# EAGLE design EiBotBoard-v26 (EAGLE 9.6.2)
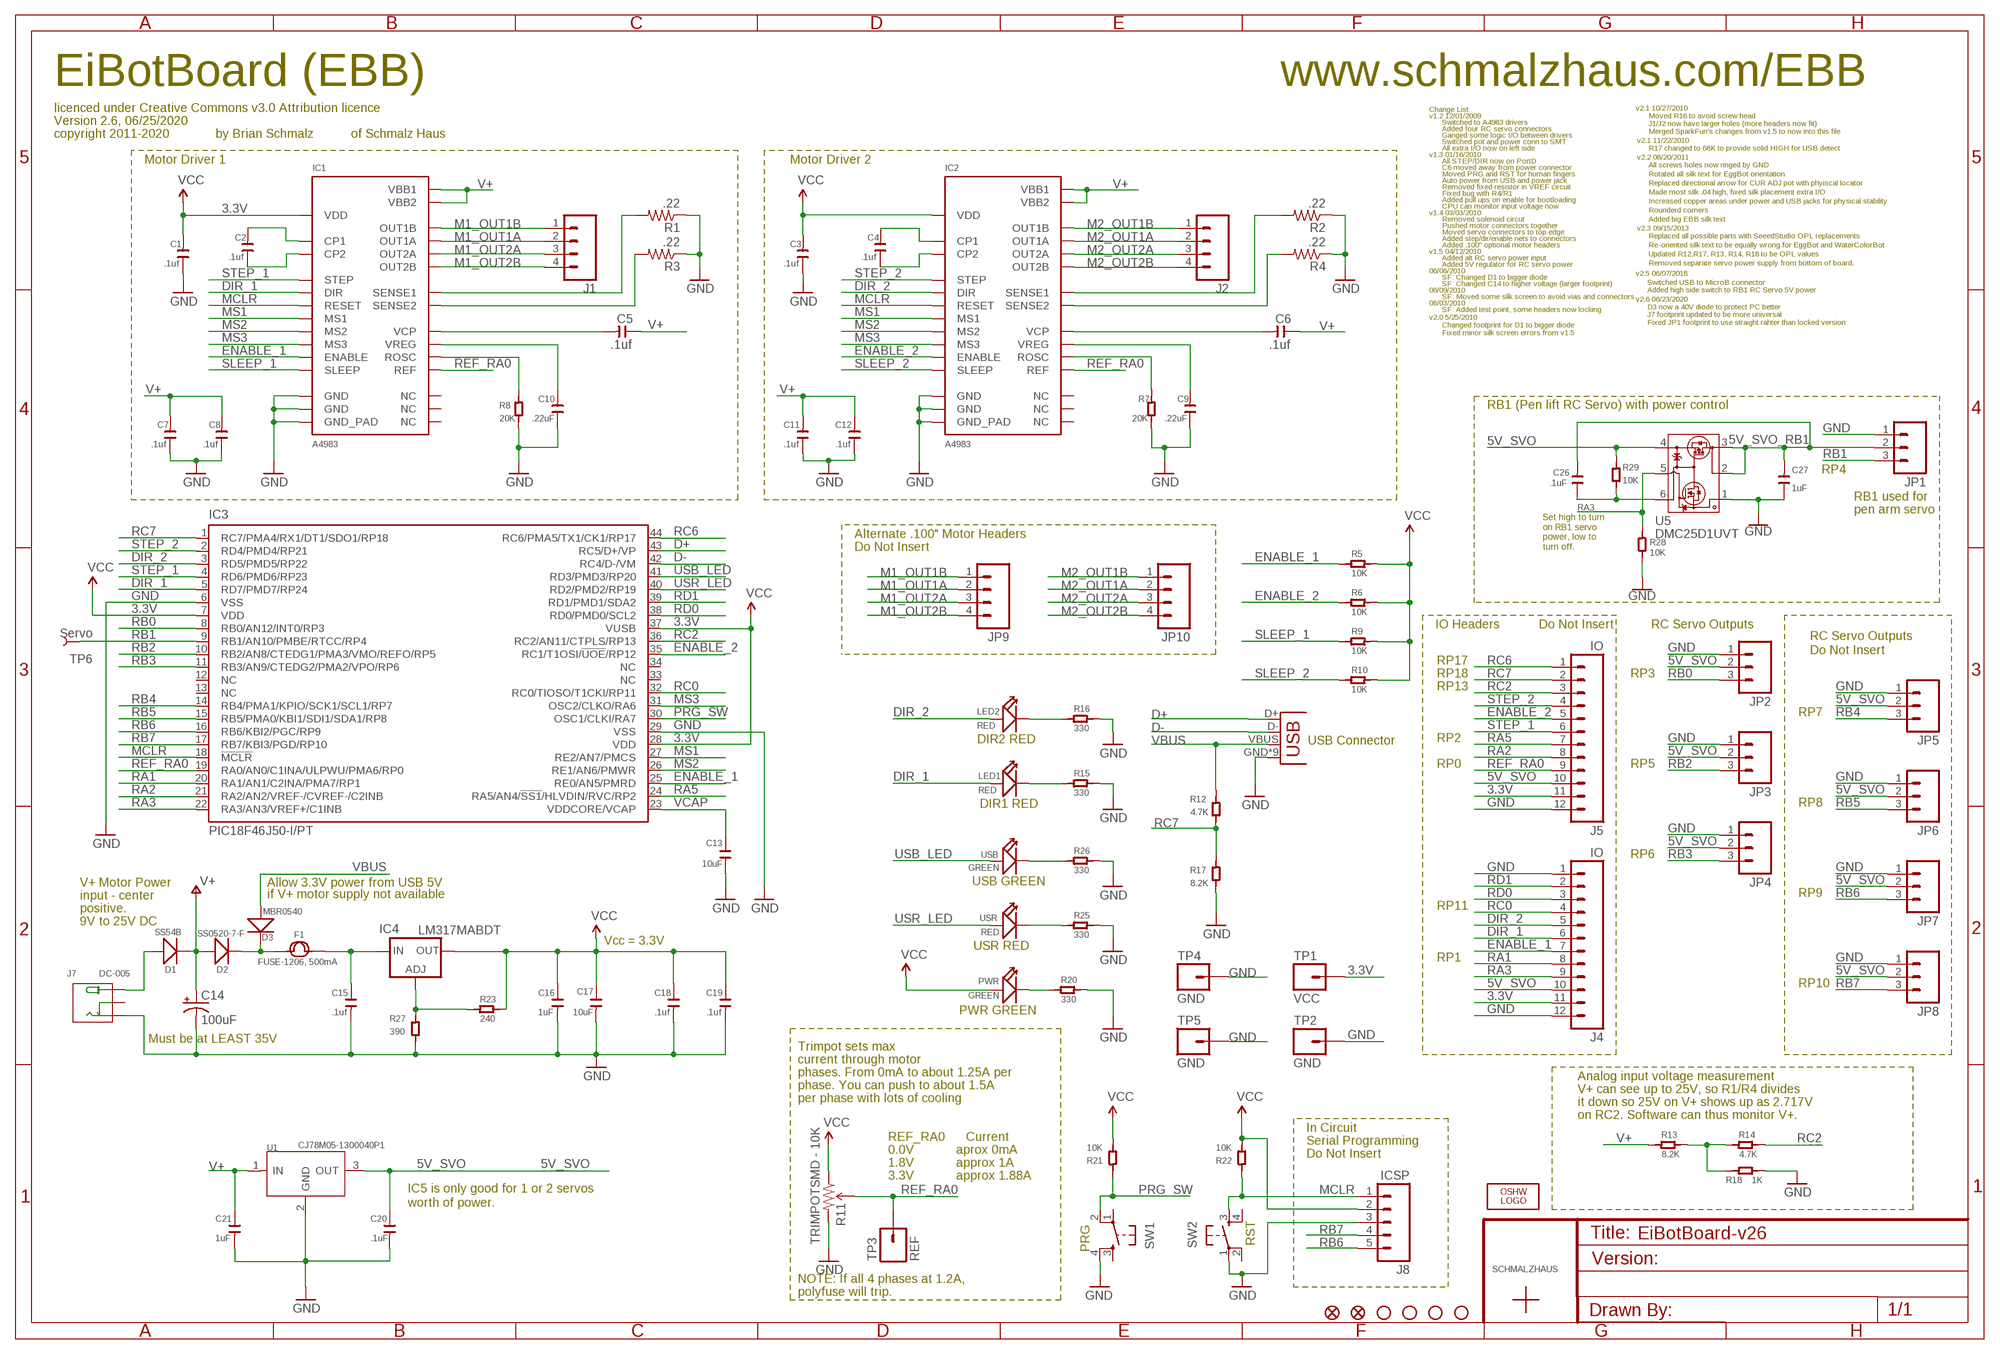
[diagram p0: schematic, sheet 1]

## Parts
C1  .1uf  C-0603  [C0603]
C2  .1uf  C-0603  [C0603]
C3  .1uf  C-0603  [C0603]
C4  .1uf  C-0603  [C0603]
C5  .1uf  C-0603  [C0603]
C6  .1uf  C-0603  [C0603]
C7  .1uf  C-0603  [C0603]
C8  .1uf  C-0603  [C0603]
C9  .22uF  C-0603  [C0603]
C10  .22uF  C-0603  [C0603]
C11  .1uf  C-0603  [C0603]
C12  .1uf  C-0603  [C0603]
C13  10uF  C-0805  [C0805]
C14  100uF  CAP_POLD  [PANASONIC_D]
C15  .1uf  C-0603  [C0603]
C16  1uF  C-0603  [C0603]
C17  10uF  C-0805  [C0805]
C18  .1uf  C-0603  [C0603]
C19  .1uf  C-0603  [C0603]
C20  .1uF  C-0603  [C0603]
C21  1uF  C-0603  [C0603]
C26  .1uF  C-0603  [C0603]
C27  1uF  C-0603  [C0603]
D1  SS54B  D-SMB  [SMB]
D2  SS0520-7-F  D-SOD-123  [SOD123]
D3  MBR0540  D-SOD-123  [SOD123]
F1  FUSE-1206, 500mA  FUSE-1206  [F1206]
IC1  A4983  [QFN28]
IC2  A4983  [QFN28]
IC3  PIC18F46J50-I/PT  PIC18F4J50  [TQFP44]
IC4  LM317MABDT  [DPACK]
J1  SCHMALZHAUS_M04  [SCHMALZHAUS_SCREWTERMINAL-3.5MM-4_LOCK]
J2  SCHMALZHAUS_M04  [SCHMALZHAUS_SCREWTERMINAL-3.5MM-4_LOCK]
J3  USBMICROB  [USB-MICROB_FCI_PINS]
J4  IO  M12PTH  [1X12]
J5  IO  M12PTH  [1X12]
J7  DC-005  CONN-POWER-JACK-2.1MM(DC-005)  [DCJ3P-14.2X11.0X9.0MM]
J8  ICSP  M05_WIDENOSILK  [1X05_NOSILK]
JP1  M031X03_NO_SILK  [1X03_NO_SILK]
JP2  M031X03_NO_SILK  [1X03_NO_SILK]
JP3  M031X03_NO_SILK  [1X03_NO_SILK]
JP4  M031X03_NO_SILK  [1X03_NO_SILK]
JP5  M031X03_NO_SILK  [1X03_NO_SILK]
JP6  M031X03_NO_SILK  [1X03_NO_SILK]
JP7  M031X03_NO_SILK  [1X03_NO_SILK]
JP8  M031X03_NO_SILK  [1X03_NO_SILK]
JP9  M04POLAR  [MOLEX-1X4]
JP10  M04POLAR  [MOLEX-1X4]
JP14  FIDUCIAL1X2  [FIDUCIAL-1X2]
JP15  FIDUCIAL1X2  [FIDUCIAL-1X2]
LED1  RED  LED  [LED0603]
LED2  RED  LED  [LED0603]
LOGO1  OSHW_LOGO_8MILX0100-NT  [OSHW_8X100_NOTEXT]
PWR  GREEN  LED  [LED0603]
R1  .22  R-US_R0805  [R0805]
R2  .22  R-US_R0805  [R0805]
R3  .22  R-US_R0805  [R0805]
R4  .22  R-US_R0805  [R0805]
R5  10K  R-0603  [R0603]
R6  10K  R-0603  [R0603]
R7  20K  R-0603  [R0603]
R8  20K  R-0603  [R0603]
R9  10K  R-0603  [R0603]
R10  10K  R-0603  [R0603]
R11  TRIMPOTSMD - 10K  TRIMPOTSMD  [TRIMPOT-3MM]
R12  4.7K  R-0603  [R0603]
R13  8.2K  R-0603  [R0603]
R14  4.7K  R-0603  [R0603]
R15  330  R-0603  [R0603]
R16  330  R-0603  [R0603]
R17  8.2K  R-0603  [R0603]
R18  1K  R-0603  [R0603]
R20  330  R-0603  [R0603]
R21  10K  R-0603  [R0603]
R22  10K  R-0603  [R0603]
R23  240  R-0603  [R0603]
R25  330  R-0603  [R0603]
R26  330  R-0603  [R0603]
R27  390  R-0603  [R0603]
R28  10K  R-0603  [R0603]
R29  10K  R-0603  [R0603]
SW1  PRG  TAC_SWITCHSND  [TACTILE_SWITCH_SMD]
SW2  RST  TAC_SWITCHSND  [TACTILE_SWITCH_SMD]
TP1  VCC  M01_WIDENOSLIK  [1X01_NOSILK]
TP2  GND  M01_WIDENOSLIK  [1X01_NOSILK]
TP3  REF  M01PTH  [1X01]
TP4  GND  M01_WIDENOSLIK  [1X01_NOSILK]
TP5  GND  M01_WIDENOSLIK  [1X01_NOSILK]
TP6  Servo  TEST-POINT3X5  [PAD.03X.05]
U1  CJ78M05-1300040P1  [TO252]
U5  DMC25D1UVT  [TSOT26]
U$1  SCHMALZHAUSSCHMALZHAUS_SMALL  [SCHMALZHAUS_SMALL]
U$2  STAND-OFF  [STAND-OFF]
U$3  STAND-OFF  [STAND-OFF]
U$4  STAND-OFF  [STAND-OFF]
U$5  STAND-OFF  [STAND-OFF]
USB  GREEN  LED  [LED0603]
USR  RED  LED  [LED0603]

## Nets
3.3V: C1.1 C3.1 C16.2 C17.2 C18.2 C19.2 IC1.P$15(VDD) IC2.P$15(VDD) IC3.7(VDD) IC3.28(VDD) IC3.37(VUSB) IC4.4(OUT) J4.11 J5.11 J8.2 PWR.+ R5.1 R6.1 R9.1 R10.1 R11.1(CCW) R21.2 R22.2 R23.2 TP1.1 ; supply symbol labelled VCC
5V_SVO: C20.2 J4.10 J5.10 JP2.2 JP3.2 JP4.2 JP5.2 JP6.2 JP7.2 JP8.2 R29.1 U1.3(OUT) U5.4(VIN_R1)
5V_SVO_RB1: C26.1 C27.1 JP1.2 U5.2(VOUT_C1$2) U5.3(VOUT_C1$1)
D+: IC3.43(RC5/D+/VP) J3.D+
D-: IC3.42(RC4/D-/VM) J3.D-
DIR_1: IC1.P$19(DIR) IC3.5(RD7/PMD7/RP24) J4.6 LED1.+
DIR_2: IC2.P$19(DIR) IC3.3(RD5/PMD5/RP22) J4.5 LED2.+
ENABLE_1: IC1.P$2(ENABLE) IC3.25(RE0/AN5/PMRD) J4.7 R5.2
ENABLE_2: IC2.P$2(ENABLE) IC3.35(RC1/T1OSI/!UOE!/RP12) J5.5 R6.2
GND: C1.2 C3.2 C7.2 C8.2 C9.2 C10.2 C11.2 C12.2 C13.1 C14.- C15.1 C16.1 C17.1 C18.1 C19.1 C20.1 C21.1 C27.2 IC1.P$3(GND) IC1.P$18(GND) IC1.P$29(GND_PAD) IC2.P$3(GND) IC2.P$18(GND) IC2.P$29(GND_PAD) IC3.6(VSS) IC3.29(VSS) J3.GND J3.GND@1(GND) J3.GND@2(GND) J3.GND@3(GND) J3.GND@4(GND) J3.GND@5(GND) J3.GND@6(GND) J3.GND@7(GND) J3.GND@8(GND) J4.1 J4.12 J5.12 J7.P$2(-) J8.3 JP1.1 JP2.1 JP3.1 JP4.1 JP5.1 JP6.1 JP7.1 JP8.1 R1.1 R2.1 R3.1 R4.1 R7.2 R8.2 R11.3(CW) R15.1 R16.1 R17.2 R18.2 R20.1 R25.1 R26.1 R27.2 R28.2 SW1.4 SW2.1 TP2.1 TP4.1 TP5.1 U1.2(GND) U5.1(R2)
M1_OUT1A: IC1.P$24(OUT1A) J1.2 JP9.2
M1_OUT1B: IC1.P$21(OUT1B) J1.1 JP9.1
M1_OUT2A: IC1.P$26(OUT2A) J1.3 JP9.3
M1_OUT2B: IC1.P$1(OUT2B) J1.4 JP9.4
M2_OUT1A: IC2.P$24(OUT1A) J2.2 JP10.2
M2_OUT1B: IC2.P$21(OUT1B) J2.1 JP10.1
M2_OUT2A: IC2.P$26(OUT2A) J2.3 JP10.3
M2_OUT2B: IC2.P$1(OUT2B) J2.4 JP10.4
MCLR: IC1.P$12(RESET) IC2.P$12(RESET) IC3.18(!MCLR!) J8.1 R22.1 SW2.3
MS1: IC1.P$9(MS1) IC2.P$9(MS1) IC3.27(RE2/AN7/PMCS)
MS2: IC1.P$10(MS2) IC2.P$10(MS2) IC3.26(RE1/AN6/PMWR)
MS3: IC1.P$11(MS3) IC2.P$11(MS3) IC3.31(OSC2/CLKO/RA6)
N$1: LED2.- R16.2
N$2: D2.- D3.- F1.1
N$3: C2.1 IC1.P$4(CP1)
N$4: R13.2 R14.1 R18.1
N$5: C2.2 IC1.P$5(CP2)
N$6: D1.+ J7.P$1(+)
N$7: LED1.- R15.2
N$8: R26.2 USB.-
N$9: IC4.1(ADJ) R23.1 R27.1
N$10: R25.2 USR.-
N$11: PWR.- R20.2
N$16: C4.1 IC2.P$4(CP1)
N$17: C4.2 IC2.P$5(CP2)
N$19: IC1.P$13(ROSC) R8.1
N$20: C10.1 IC1.P$8(VREG)
N$21: C5.1 IC1.P$6(VCP)
N$31: IC1.P$27(SENSE2) R3.2
N$32: IC1.P$23(SENSE1) R1.2
N$36: C15.2 F1.2 IC4.3(IN)
N$41: C6.1 IC2.P$6(VCP)
N$43: IC2.P$23(SENSE1) R2.2
N$44: IC2.P$27(SENSE2) R4.2
N$45: C9.1 IC2.P$8(VREG)
N$48: IC2.P$13(ROSC) R7.1
N$1234: C26.2 R29.2 U5.6(R1_C1)
PRG_SW: IC3.30(OSC1/CLKI/RA7) R21.1 SW1.2
RA1: IC3.20(RA1/AN1/C2INA/PMA7/RP1) J4.8
RA2: IC3.21(RA2/AN2/VREF-/CVREF-/C2INB) J5.8
RA3: IC3.22(RA3/AN3/VREF+/C1INB) J4.9 R28.1 U5.5(ON/OFF)
RA5: IC3.24(RA5/AN4/!SS1!/HLVDIN/RVC/RP2) J5.7
RB0: IC3.8(RB0/AN12/INT0/RP3) JP2.3
RB1: IC3.9(RB1/AN10/PMBE/RTCC/RP4) JP1.3 TP6.P$1
RB2: IC3.10(RB2/AN8/CTEDG1/PMA3/VMO/REFO/RP5) JP3.3
RB3: IC3.11(RB3/AN9/CTEDG2/PMA2/VPO/RP6) JP4.3
RB4: IC3.14(RB4/PMA1/KPIO/SCK1/SCL1/RP7) JP5.3
RB5: IC3.15(RB5/PMA0/KBI1/SDI1/SDA1/RP8) JP6.3
RB6: IC3.16(RB6/KBI2/PGC/RP9) J8.5 JP7.3
RB7: IC3.17(RB7/KBI3/PGD/RP10) J8.4 JP8.3
RC0: IC3.32(RC0/TIOSO/T1CKI/RP11) J4.4
RC2: IC3.36(RC2/AN11/CTPLS/RP13) J5.3 R14.2
RC6: IC3.44(RC6/PMA5/TX1/CK1/RP17) J5.1
RC7: IC3.1(RC7/PMA4/RX1/DT1/SDO1/RP18) J5.2 R12.2 R17.1
RD0: IC3.38(RD0/PMD0/SCL2) J4.3
RD1: IC3.39(RD1/PMD1/SDA2) J4.2
REF_RA0: IC1.P$17(REF) IC2.P$17(REF) IC3.19(RA0/AN0/C1INA/ULPWU/PMA6/RP0) J5.9 R11.2(WIPER) TP3.1
SLEEP_1: IC1.P$14(SLEEP) R9.2
SLEEP_2: IC2.P$14(SLEEP) R10.2
STEP_1: IC1.P$16(STEP) IC3.4(RD6/PMD6/RP23) J5.6
STEP_2: IC2.P$16(STEP) IC3.2(RD4/PMD4/RP21) J5.4
USB_LED: IC3.41(RD3/PMD3/RP20) USB.+
USR_LED: IC3.40(RD2/PMD2/RP19) USR.+
V+: C5.2 C6.2 C7.1 C8.1 C11.1 C12.1 C14.+ C21.2 D1.- D2.+ IC1.P$22(VBB1) IC1.P$28(VBB2) IC2.P$22(VBB1) IC2.P$28(VBB2) R13.1 U1.1(IN)
VBUS: D3.+ J3.VBUS R12.1
VCAP: C13.2 IC3.23(VDDCORE/VCAP)
Unconnected: IC1.P$7(NC) IC1.P$20(NC) IC1.P$25(NC) IC2.P$7(NC) IC2.P$20(NC) IC2.P$25(NC) IC3.12(NC) IC3.13(NC) IC3.33(NC) IC3.34(NC) J7.P$3(CDN) SW1.1 SW1.3 SW2.2 SW2.4

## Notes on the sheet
- EiBotBoard (EBB) | www.schmalzhaus.com/EBB
- licenced under Creative Commons v3.0 Attribution licence | Change List | v2.1 10/27/2010
- v1.2 12/01/2009 | Moved R16 to avoid screw head
- Version 2.6, 06/25/2020 | Switched to A4983 drivers | J1/J2 now have larger holes (more headers now fit)
- Added four RC servo connectors
- Merged SparkFun's changes from v1.5 to now into this file
- copyright 2011-2020 | by Brian Schmalz | of Schmalz Haus | Ganged some logic I/O between drivers
- Switched pot and power conn to SMT | v2.1 11/22/2010
- All extra I/O now on left side | R17 changed to 68K to provide solid HIGH for USB detect
- v1.3 01/16/2010
- v2.2 08/20/2011
- Motor Driver 1 | Motor Driver 2 | All STEP/DIR now on PortD
- All screws holes now ringed by GND
- C6 moved away from power connector
- Moved PRG and RST for human fingers | Rotated all silk text for EggBot orientation
- Auto power from USB and power jack
- Replaced directional arrow for CUR ADJ pot with phyiscal locator
- Removed fixed resistor in VREF circuit
- Fixed bug with R4/R1 | Made most silk .04 high, fixed silk placement extra I/O
- Added pull ups on enable for bootloading | Increased copper areas under power and USB jacks for physical stability
- CPU can monitor input voltage now
- Rounderd corners
- v1.4 03/03/2010
- Removed solenoid circut | Added big EBB silk text
- Pushed motor connectors together
- v2.3 09/15/2013
- Moved servo connectors to top edge
- Replaced all possible parts with SeeedStudio OPL replacements
- Added step/dir/enable nets to connectors
- Added .100" optional motor headers | Re-oriented silk text to be equally wrong for EggBot and WaterColorBot
- v1.5 04/12/2010
- Updated R12,R17, R13, R14, R18 to be OPL values
- Added alt RC servo power input
- Added 5V regulator for RC servo power | Removed separate servo power supply from bottom of board.
- 06/06/2010
- v2.5 06/07/2018
- SF: Changed D1 to bigger diode
- SF: Changed C14 to higher voltage (larger footprint)
- 06/09/2010
- Switched USB to MicroB connector
  Added high side switch to RB1 RC Servo 5V power
- SF: Moved some silk screen to avoid vias and connectors
- v2.6 06/23/2020
- 08/03/2010
- SF: Added test point, some headers now locking
- v2.0 5/25/2010
- D3 now a 40V diode to protect PC better
  J7 footprint updated to be more universal
  Fixed JP1 footprint to use straight rahter than locked version
- Changed footprint for D1 to bigger diode
- Fixed minor silk screen errors from v1.5
- RB1 (Pen lift RC Servo) with power control
- RP4
- RB1 used for
- pen arm servo
- Alternate .100" Motor Headers
- Set high to turn 
  on RB1 servo 
  power, low to 
  turn off.
- Do Not Insert
- IO Headers | Do Not Insert | RC Servo Outputs
- RC Servo Outputs
- Do Not Insert
- RP17
- RP18 | RP3
- RP13
- RP7
- DIR2 RED | USB Connector | RP2
- RP0 | RP5
- DIR1 RED | RP8
- RP6
- V+ Motor Power | Allow 3.3V power from USB 5V | USB GREEN
- input - center | if V+ motor supply not available | RP9
- positive. | RP11
- 9V to 25V DC
- Vcc = 3.3V
- USR RED
- RP1
- RP10
- PWR GREEN
- Must be at LEAST 35V
- Trimpot sets max
- current through motor
- phases. From 0mA to about 1.25A per
- Analog input voltage measurement
- phase. You can push to about 1.5A
- V+ can see up to 25V, so R1/R4 divides
- per phase with lots of cooling
- it down so 25V on V+ shows up as 2.717V
- on RC2. Software can thus monitor V+.
- In Circuit
- REF_RA0      Current
- Serial Programming
- 0.0V            aprox 0mA
- Do Not Insert
- 1.8V            approx 1A
- 3.3V            approx 1.88A
- IC5 is only good for 1 or 2 servos
- worth of power.
- PRG
- RST
- NOTE: If all 4 phases at 1.2A,
- polyfuse will trip.

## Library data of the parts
C1-C13 C15-C21 C26 C27 = OPL Eagle Library:C*
C14 = SparkFun:CAP_POL: Capacitor Polarized
D1-D3 = OPL Eagle Library:D*: DIODE
F1 = OPL Eagle Library:FUSE*
IC1 IC2 = SchmalzHaus:A4983
IC3 = SchmalzHaus:PIC18F4*J50
IC4 = v-reg:LM317?*: 500 mA Adjustable Output Positive Voltage Regulator Source: http://www.onsemi.co.jp .. LM317M-D.PDF
J1 J2 = EiBotBoard-v21:SCHMALZHAUS_M04: Header 4 Standard 4-pin 0.1" header. Use with straight break away headers (SKU : PRT-00116), right angle break away headers (PRT-00553), swiss pins (PRT-00743), machine pins (PRT-00117), and female headers (PRT-00115). Molex polarized connector foot print use with SKU : PRT-08231 with associated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
J3 = SchmalzHaus:USB: USB Connectors USB-B-PTH is fully proven SKU : PRT-00139 USB-miniB is fully proven SKU : PRT-00587 USB-A-PCB is untested. USB-A-H is throughly reviewed, but untested. Spark Fun Electronics SKU : PRT-00437 USB-B-SMT is throughly reviewed, but untested. Needs silkscreen touching up. USB-A-S has not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
J4 J5 = SparkFun-12-01-09:M12: Header 12 Standard 12-pin 0.1" header. Use with straight break away headers (SKU : PRT-00116), right angle break away headers (PRT-00553), swiss pins (PRT-00743), machine pins (PRT-00117), and female headers (PRT-00115).
J7 = OPL_Connector_SH:CONN-POWER-JACK-2.1MM(DC-005): Seeed SKU 320120003 - DIP Black DC Jack 2.1MM MPN: DC-005 Important Notes: This part requires milling slots. Please make sure layer 46 Milling is included in the profile or outline layer when exporting Gerber files. Alternatively, you can use the built-in Seeed Fusion CAM file. Find it under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; MPN: DC-005
J8 = SchmalzHaus:M05_WIDE: Header 5 Standard 5-pin 0.1" header. Use with straight break away headers (SKU : PRT-00116), right angle break away headers (PRT-00553), swiss pins (PRT-00743), machine pins (PRT-00117), and female headers (PRT-00115). Molex polarized connector foot print use with SKU : PRT-08230 with associated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
JP1 = SparkFun:M03: Header 3 Standard 3-pin 0.1" header. Use with straight break away headers (SKU : PRT-00116), right angle break away headers (PRT-00553), swiss pins (PRT-00743), machine pins (PRT-00117), and female headers (PRT-00115). Molex polarized connector foot print use with SKU : PRT-08232 with associated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
JP2-JP8 = SparkFun-12-01-09:M03: Header 3 Standard 3-pin 0.1" header. Use with straight break away headers (SKU : PRT-00116), right angle break away headers (PRT-00553), swiss pins (PRT-00743), machine pins (PRT-00117), and female headers (PRT-00115). Molex polarized connector foot print use with SKU : PRT-08232 with associated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
JP9 JP10 = SparkFun-12-01-09:M04: Header 4 Standard 4-pin 0.1" header. Use with straight break away headers (SKU : PRT-00116), right angle break away headers (PRT-00553), swiss pins (PRT-00743), machine pins (PRT-00117), and female headers (PRT-00115). Molex polarized connector foot print use with SKU : PRT-08231 with associated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
JP14 JP15 = SparkFun:FIDUCIAL: Fiducial Alignment Points
LED1 LED2 PWR USB USR = OPL Eagle Library:LED*: LED
LOGO1 = OSHW:OSHW_LOGO_8MIL
R1-R4 = rcl:R-US_: RESISTOR, American symbol; SPICEPREFIX: R
R5-R10 R12-R18 R20-R23 R25-R29 = OPL Eagle Library:R*
R11 = SparkFun11_03_09:TRIMPOT
SW1 SW2 = SparkFunEagle-6-6-07:TAC_SWITCH: Momentary Switch Button commonly used for reset or general input. Spark Fun Electronics SKU : COM-00097
TP1 TP2 TP4 TP5 = SchmalzHaus:M01_WIDE: Header 1
TP3 = SchmalzHaus:M01: Header 1
TP6 = SparkFun:TEST-POINT
U1 = OPL Eagle Library:CJ78M05: 0.5A Three Terminal Positive Voltage Regulators
U5 = DiodesInc_DMC25D1UVT:DMC25D1UVT: Diodes Incorporated DMC25D1UVT.
U$1 = SchmalzHaus:SCHMALZHAUS
U$2-U$5 = SparkFun01082009:STAND-OFF: Stand Off

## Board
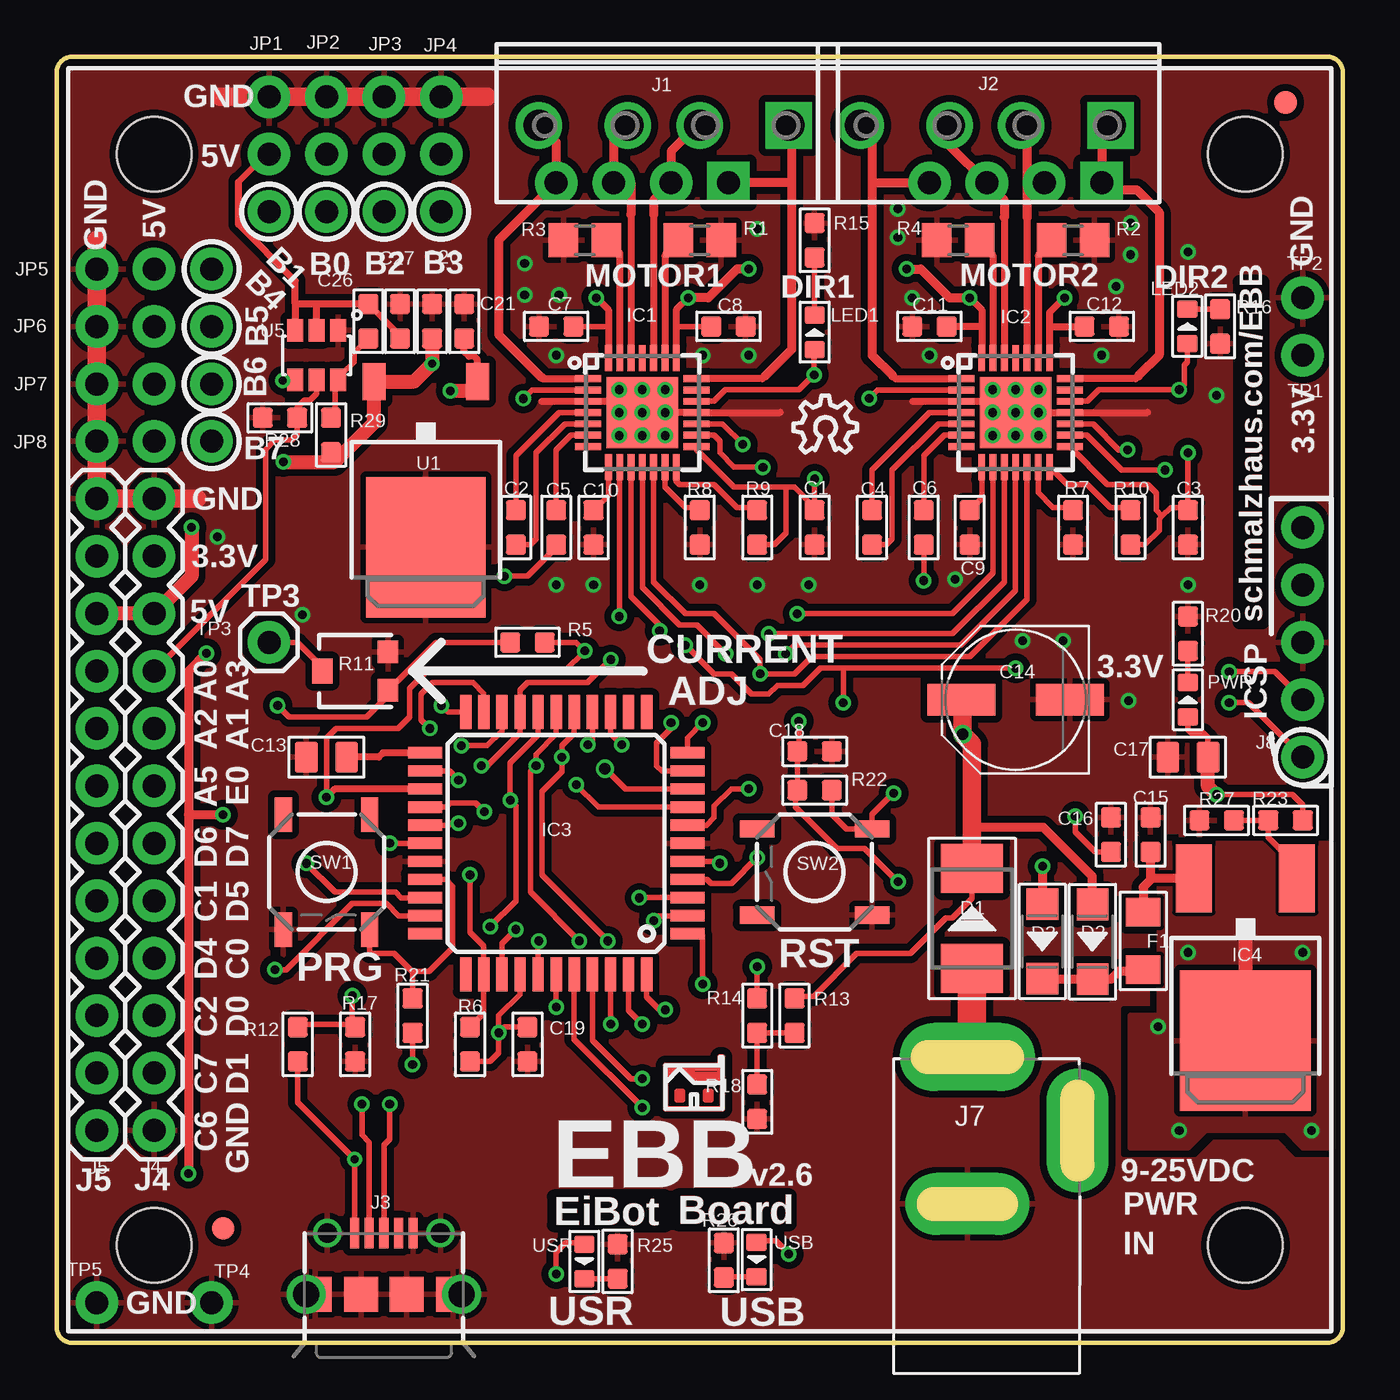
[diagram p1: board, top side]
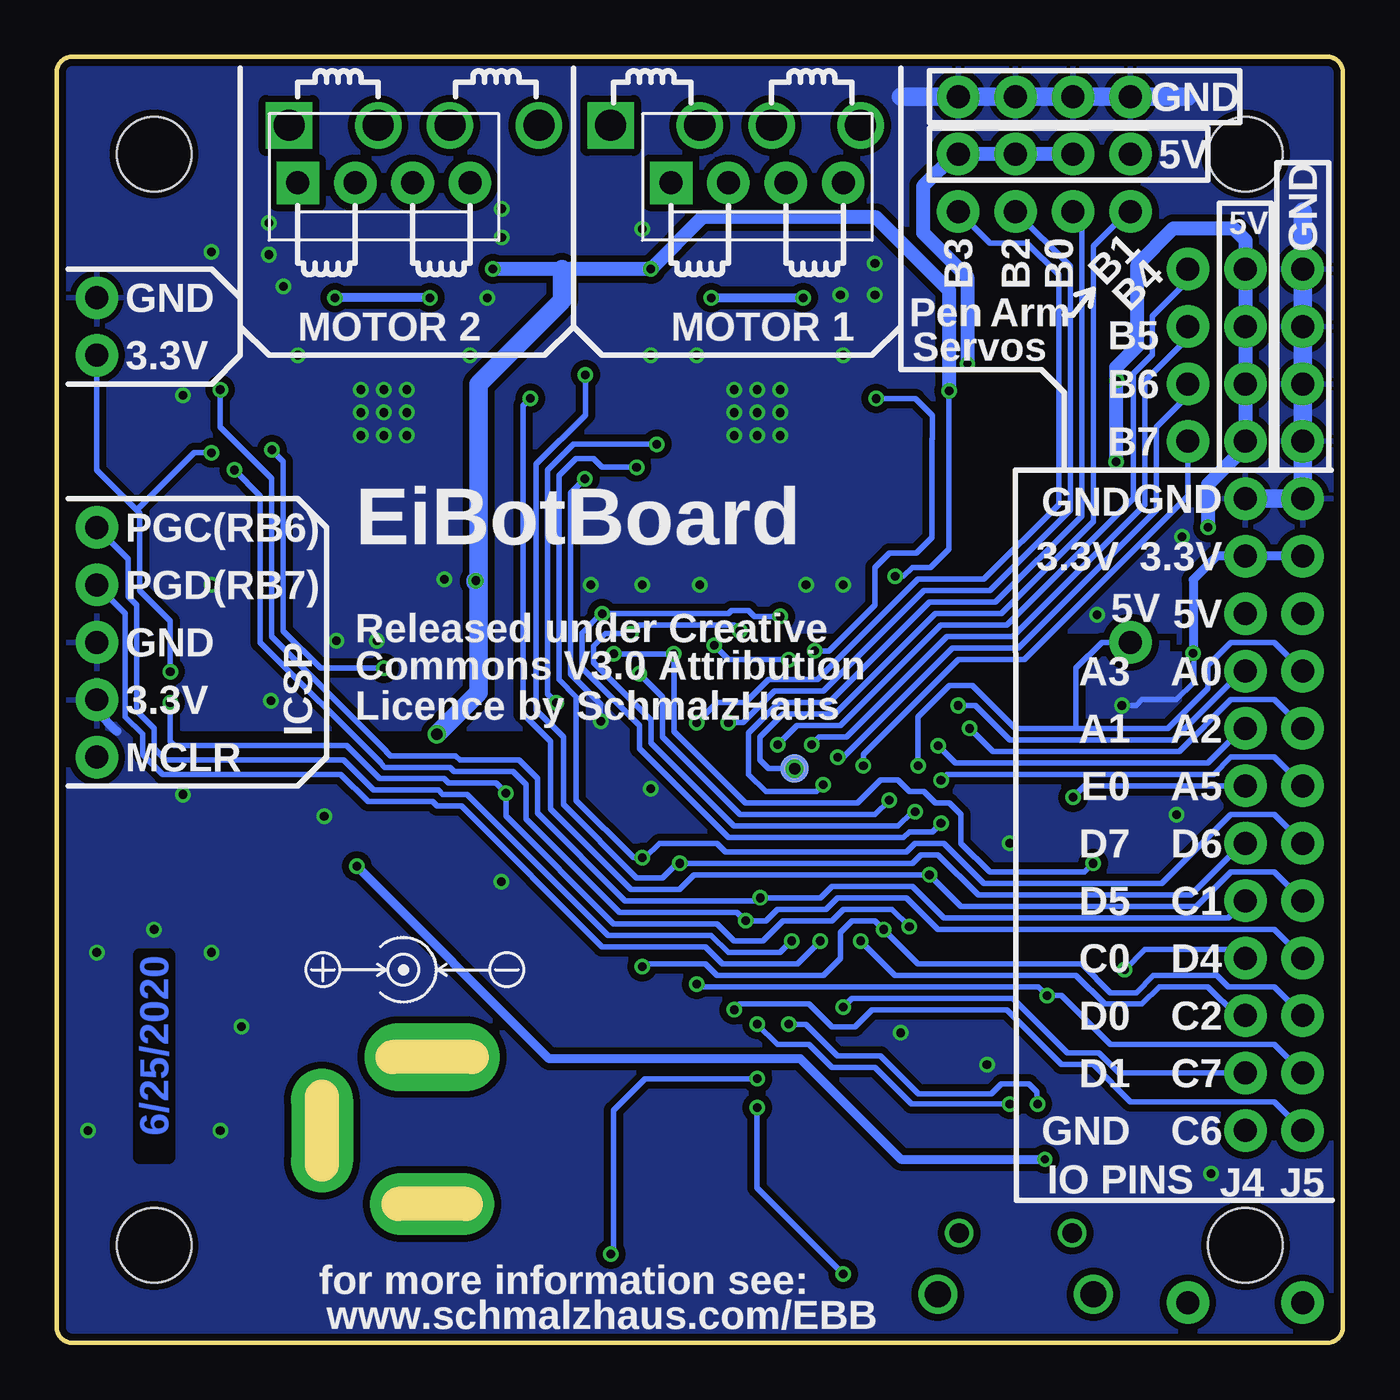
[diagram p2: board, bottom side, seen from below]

Size 56.9 x 56.9 mm. Coordinates in mm from the lower left corner, seen from the top.
Outline: 56.18,0 arc90 56.9,0.72 56.9,56.18 arc90 56.18,56.9 0.72,56.9 arc90 0,56.18 0,0.72 arc90 0.72,0 56.18,0
Copper layers (1*16): Top 0.035mm / dielectric 0.2mm / Bottom 0.035mm
Design rules "SeeedStudio_DRU_20130527 *": minimum track width 6mil, minimum drill 12mil, track to track 6mil, track to pad 6mil, pad to pad 6mil, via to via 6mil, smd to smd 0mil, copper to edge 10mil, drill to drill 10mil, minimum pad ring 6mil, minimum via ring 6mil, stop-mask expansion 2mil, vias tented up to drill 25mil, thermal gap 10mil

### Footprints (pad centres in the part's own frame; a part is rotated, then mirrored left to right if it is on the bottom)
C0603 = smd 0.889 x 0.889: 1 -0.762,0; 2 0.762,0
C0805 = smd 1.016 x 1.397: 1 -0.889,0; 2 0.889,0
PANASONIC_D = smd 3 x 1.4: + 2.4,0; - -2.4,0
SMB = smd 2.159 x 2.743: + -2.21,0; - 2.21,0
SOD123 = smd 1.397 x 1.397: + -1.651,0; - 1.651,0
F1206 = smd 1.27 x 1.524: 1 -1.27,0; 2 1.27,0
QFN28 = smd 1.15 x 0.3: P$1 -2.4,1.5; P$2 -2.4,1; P$3 -2.4,0.5; P$4 -2.4,0; P$5 -2.4,-0.5; P$6 -2.4,-1; P$7 -2.4,-1.5; P$15 2.4,-1.5; P$16 2.4,-1; P$17 2.4,-0.5; P$18 2.4,0; P$19 2.4,0.5; P$20 2.4,1; P$21 2.4,1.5 | smd 0.3 x 1.15: P$8 -1.5,-2.4; P$9 -1,-2.4; P$10 -0.5,-2.4; P$11 0,-2.4; P$12 0.5,-2.4; P$13 1,-2.4; P$14 1.5,-2.4; P$22 1.5,2.4; P$23 1,2.4; P$24 0.5,2.4; P$25 0,2.4; P$26 -0.5,2.4; P$27 -1,2.4; P$28 -1.5,2.4 | smd 3.15 x 3.15: P$29 0,0
TQFP44 = smd 1.5 x 0.5: 1 -5.8,4; 2 -5.8,3.2; 3 -5.8,2.4; 4 -5.8,1.6; 5 -5.8,0.8; 6 -5.8,0; 7 -5.8,-0.8; 8 -5.8,-1.6; 9 -5.8,-2.4; 10 -5.8,-3.2; 11 -5.8,-4; 23 5.8,-4; 24 5.8,-3.2; 25 5.8,-2.4; 26 5.8,-1.6; 27 5.8,-0.8; 28 5.8,0; 29 5.8,0.8; 30 5.8,1.6; 31 5.8,2.4; 32 5.8,3.2; 33 5.8,4 | smd 0.5 x 1.5: 12 -4,-5.8; 13 -3.2,-5.8; 14 -2.4,-5.8; 15 -1.6,-5.8; 16 -0.8,-5.8; 17 0,-5.8; 18 0.8,-5.8; 19 1.6,-5.8; 20 2.4,-5.8; 21 3.2,-5.8; 22 4,-5.8; 34 4,5.8; 35 3.2,5.8; 36 2.4,5.8; 37 1.6,5.8; 38 0.8,5.8; 39 0,5.8; 40 -0.8,5.8; 41 -1.6,5.8; 42 -2.4,5.8; 43 -3.2,5.8; 44 -4,5.8
DPACK = smd 1.6 x 3: 1 -2.28,-4.8; 3 2.28,-4.8 | smd 5.8 x 6.2: 4 0,2.38
SCHMALZHAUS_SCREWTERMINAL-3.5MM-4_LOCK = drill 1.372 square: 1 -0.127,0 | drill 1.372: 2 3.81,0; 3 6.985,0; 4 10.922,0
USB-MICROB_FCI_PINS = smd 0.4 x 1.35: D+ 0,2.7; D- -0.65,2.7; GND 1.3,2.7; ID 0.65,2.7; VBUS -1.3,2.7 | drill 1.15: GND@1 -3.445,0; GND@2 3.445,0 | drill 0.85: GND@3 -2.5,2.7; GND@4 2.5,2.7 | smd 1.5 x 1.55: GND@5 -3.05,0; GND@6 -1,0; GND@7 1,0; GND@8 3.05,0
1X12 = drill 1.016 pad 1.88: 1 0,0; 2 2.54,0; 3 5.08,0; 4 7.62,0; 5 10.16,0; 6 12.7,0; 7 15.24,0; 8 17.78,0; 9 20.32,0; 10 22.86,0; 11 25.4,0; 12 27.94,0
DCJ3P-14.2X11.0X9.0MM = drill 0.6 pad 3 long: P$1 3.25,0 | drill 0.6 pad 2.75 long: P$2 -3.25,0; P$3 0,-4.877
1X05_NOSILK = drill 1.016 pad 1.88: 1 0,0; 2 2.54,0; 3 5.08,0; 4 7.62,0; 5 10.16,0
1X03_NO_SILK = drill 1.016 pad 1.88: 1 0,0; 2 2.54,0; 3 5.08,0
MOLEX-1X4 = drill 1.016 pad 1.88 square: 1 0,0 | drill 1.016 pad 1.88: 2 2.54,0; 3 5.08,0; 4 7.62,0
FIDUCIAL-1X2 = smd 1 x 1: 1 0,0
LED0603 = smd 0.762 x 0.889: + -0.762,0; - 0.762,0
R0805 = smd 1.3 x 1.5: 1 -0.95,0; 2 0.95,0
R0603 = smd 0.889 x 0.889: 1 -0.762,0; 2 0.762,0
TRIMPOT-3MM = smd 1 x 0.9: 1 -0.85,-1.45; 3 0.85,-1.45 | smd 1.1 x 0.9: 2 0,1.45
TACTILE_SWITCH_SMD = smd 1.524 x 0.762: 1 -2.54,1.905; 2 2.54,1.905; 3 -2.54,-1.905; 4 2.54,-1.905
1X01_NOSILK = drill 1.016 pad 1.88: 1 0,0
1X01 = drill 1.016 pad 1.88: 1 0,0
PAD.03X.05 = smd 1.27 x 1.27: P$1 0,0
TO252 = smd 1.016 x 1.651: 1 -2.286,-4.826; 3 2.286,-4.826 | smd 5.3 x 6.2: 2 0,2.5
TSOT26 = smd 0.7 x 1: 1 -0.95,-1.099; 2 0,-1.099; 3 0.95,-1.099; 4 0.95,1.099; 5 0,1.099; 6 -0.95,1.099
STAND-OFF = hole 3.302: 0,0

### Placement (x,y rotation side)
C1  33.53,36.07 270 top
C2  20.32,36.07 270 top
C3  50.04,36.07 270 top
C4  36.07,36.07 270 top
C5  22.1,36.07 270 top
C6  38.35,36.07 270 top
C7  22.1,44.96 180 top
C8  29.72,44.96 0 top
C9  40.39,36.07 270 top
C10  23.75,36.07 270 top
C11  38.61,44.96 180 top
C12  46.23,44.96 0 top
C13  11.94,25.91 0 top
C14  42.42,28.45 180 top
C15  48.39,22.48 270 top
C16  46.63,22.48 270 top
C17  50.04,25.91 0 top
C18  33.53,26.16 180 top
C19  20.83,13.21 90 top
C20  16.61,45.19 270 top
C21  18.03,45.19 270 top
C26  13.79,45.19 270 top
C27  15.19,45.19 90 top
D1  40.49,18.78 90 top
D2  45.82,17.75 270 top
D3  43.6,17.76 270 top
F1  48.06,17.78 90 top
IC1  25.91,41.15 0 top
IC2  42.42,41.15 0 top
IC3  22.1,22.1 180 top
IC4  52.58,15.75 180 top
J1  32.26,53.85 180 top
J2  46.48,53.85 180 top
J3  14.48,2.16 0 top
J4  4.32,9.4 90 top
J5  1.78,9.4 90 top
J7  40.28,9.4 90 top
J8  55.12,25.91 90 top
JP1  9.4,55.12 270 top
JP2  11.94,55.12 270 top
JP3  14.48,55.12 270 top
JP4  17.02,55.12 270 top
JP5  1.78,47.5 0 top
JP6  1.78,44.96 0 top
JP7  1.78,42.42 0 top
JP8  1.78,39.88 0 top
JP9  29.72,51.31 0 bottom
JP10  46.23,51.31 0 bottom
JP14  54.36,54.86 0 top
JP15  7.37,5.08 0 top
LED1  33.53,44.7 90 top
LED2  50.01,44.96 90 top
LOGO1  32.59,39.37 0 top
PWR  50.04,28.45 90 top
R1  28.45,48.77 180 top
R2  44.96,48.77 180 top
R3  23.37,48.77 0 top
R4  39.88,48.77 0 top
R5  20.83,30.99 0 top
R6  18.29,13.21 90 top
R7  44.96,36.07 270 top
R8  28.45,36.07 270 top
R9  30.99,36.07 90 top
R10  47.5,36.07 90 top
R11  13.21,29.72 90 top
R12  10.67,13.21 90 top
R13  32.64,14.48 270 top
R14  30.99,14.48 90 top
R15  33.53,48.77 270 top
R16  51.46,44.96 90 top
R17  13.21,13.21 270 top
R18  30.99,10.67 270 top
R20  50.04,31.37 270 top
R21  15.75,14.48 270 top
R22  33.53,24.45 180 top
R23  54.36,23.11 0 top
R25  24.82,3.61 270 top
R26  29.51,3.66 270 top
R27  51.31,23.11 180 top
R28  9.88,40.92 180 top
R29  12.14,40.16 90 top
SW1  11.94,20.83 270 top
SW2  33.53,20.83 180 top
TP1  55.12,43.69 0 top
TP2  55.12,46.23 0 top
TP3  9.4,30.99 0 top
TP4  6.86,1.78 0 top
TP5  1.78,1.78 0 top
TP6  24.26,25.4 0 bottom
U1  16.33,37.69 180 top
U5  11.51,43.69 180 top
U$1  28.19,10.36 0 top
U$2  52.58,4.32 0 top
U$3  4.32,4.32 0 top
U$4  52.58,52.58 0 top
U$5  4.32,52.58 0 top
USB  30.96,3.68 270 top
USR  23.34,3.61 270 top

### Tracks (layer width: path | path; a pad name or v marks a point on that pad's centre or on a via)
3.3V  (via drill 0.38)
  Top 0.254: IC1.P$15 28.31,39.51 29.97,37.85 32.26,37.85 | 32.26,37.85 32.64,37.85 33.53,36.96 C1.1 v33.53,38.23 | IC3.37 20.5,15.42 19.56,14.48 v19.56,13.72 | 48.9,36.58 48.77,36.45 48.77,35.94 48.13,35.31 R10.1 | 48.9,36.58 49.28,36.96 50,36.96 50,36.87 C3.1 v50.04,39.37 | 32.26,37.85 32.26,35.81 31.75,35.31 R9.1 | R21.2 v15.75,12.32 | v19.56,13.72 19.56,12.83 19.18,12.45 R6.1 | IC3.7 28.74,22.9 29.08,23.24 29.08,23.75 29.84,24.51 v30.61,24.51 | v14.73,22.1 IC3.28 | 48.9,36.58 48.64,36.83 48.64,37.59 48.26,37.97 46.48,37.97 44.82,39.64 IC2.P$15 | R5.1 16.78,30.99 R11.1 14.66,28.63 13.72,27.69 10.29,27.69 v9.78,28.19 | v37.22,20.4 35.74,21.88 34.49,21.88 34.49,21.89 32.69,23.7 32.69,24.44 32.7,24.45 R22.2 C18.2 32.83,26.23 v32.83,27.5 | v45.06,23.29 45.06,22.61 45.95,21.72 C16.2 | R23.2 55.12,23.8 54.66,24.26 v51.31,24.26 51.28,24.26 | C19.2 19.81,13.97 v19.56,13.72 | C17.2 50.93,26.77 50.72,26.97 50.19,26.97 50.04,27.13 PWR.+ | v51.87,29.69 53.87,29.69 J8.2
  Top 0.406: 5.84,23.37 v5.84,7.49 | 5.84,23.37 v7.37,23.37 | 5.84,23.37 5.84,29.72 v6.63,30.5
  Top 0.61: v52.58,18.29 IC4.4 | 51.28,24.26 50.93,24.61 C17.2
  Bottom 0.254: v33.53,38.23 34.16,37.59 34.16,29.59 32.83,28.26 v32.83,27.5 | v51.87,29.69 51.87,31.93 53.21,33.27 53.21,36.7 53.34,36.83 | 53.34,36.83 55.12,38.61 TP1.1 | v50.04,39.37 50.8,39.37 53.34,36.83 | v6.63,30.5 6.6,30.48 6.6,29.21 7.37,28.45 8.89,28.45 9.14,28.19 v9.78,28.19
  Bottom 0.406: J5.11 J4.11 5.59,34.8 6.63,33.76 v6.63,30.5 | J8.2 55.12,27.94 54.23,27.05
  other vias: 48.72,14 55.5,9.4 49.66,9.4 55.12,17.27 50.04,17.27
  pour Bottom (isolate 0.305, rank 3): 0.25,28.45 0.25,0.25 56.64,0.25 56.64,29.72 52.58,29.72 52.58,25.91 39.88,25.91 33.53,31.5 7.24,31.5 7.24,28.45
  pour Top: 47.5,14.48 47.5,8.64 50.04,8.64 50.8,9.4 54.36,9.4 55.12,8.64 56.39,8.64 56.39,22.1 48.77,22.1 48.77,14.48
5V_SVO  (via drill 0.35, 0.38)
  Top 0.254: U5.4 10.03,42.59 v10.01,42.56 | R29.1 12.29,39.24 12.29,38.96
  Top 0.61: v5.97,36.07 5.97,33.91 J4.10 J5.10 | v10.03,38.96 12.29,38.96 12.76,39.43 14.05,40.72 U1.3 15.82,42.52 v16.61,43.31 C20.2
  Bottom 0.254: 10.03,43.16 10.03,42.59 v10.01,42.56
  Bottom 0.406: JP8.2 4.32,39.62
  Bottom 0.61: JP2.2 JP3.2 JP4.2 17.14,52.58 18.57,51.16 18.57,49.1 16.61,47.14 v16.61,43.31 | JP8.2 JP7.2 JP6.2 JP5.2 4.32,48.77 4.85,49.3 7.49,49.3 9.09,47.7 9.09,44.09 10.03,43.16 v10.03,38.96 | 4.32,39.62 5.97,37.97 v5.97,36.07
5V_SVO_RB1
  Top 0.254: C26.1 15.19,44.55 C27.1 | 10.57,45.95 10.56,45.96 | 10.56,46.98 10.54,46.99 | 8.05,51.36 9.27,52.58 JP1.2
  Top 0.305: U5.3 10.56,45.96 10.56,46.98 | 10.54,46.99 8.05,49.48 8.05,51.36 | C26.1 11.51,45.95 | 11.51,45.95 10.57,45.95 | U5.2 11.51,45.95
D+  (via drill 0.38)
  Top 0.254: IC3.43 25.3,14.71 v25.91,14.1 | J3.D+ 14.48,8.76 14.73,9.02 v14.73,10.57
  Bottom 0.254: v25.91,14.1 25.02,13.21 23.62,13.21 22.61,12.19 20.7,12.19 19.07,10.57 v14.73,10.57
D-  (via drill 0.38)
  Top 0.254: IC3.42 24.5,14.11 v24.51,14.1 | J3.D- 13.83,8.88 13.51,9.2 v13.51,10.57
  Bottom 0.254: v24.51,14.1 23.75,14.1 22.35,12.7 20.45,12.7 18.77,11.02 15.55,11.02 15.11,11.45 13.89,11.45 13.54,11.1 13.54,10.59 v13.51,10.57
DIR_1  (via drill 0.38)
  Top 0.254: IC3.5 29.3,21.3 29.3,21.25 v29.34,21.21 | IC1.P$19 29.07,41.65 29.59,42.16 32.84,42.16 v33.5,42.82 33.5,43.69 33.53,43.71 LED1.+
  Bottom 0.254: J4.6 4.45,22.1 6.73,19.81 16.13,19.81 17.91,21.59 18.67,21.59 19.05,21.21 v29.34,21.21 29.46,21.21 30.1,20.57 31.24,20.57 34.48,23.81 34.48,26.8 35.69,28 35.69,38.86 33.5,41.05 v33.5,42.82
DIR_2  (via drill 0.38)
  Top 0.254: IC3.3 25.79,19.7 v25.78,19.68 | IC2.P$19 45.59,41.65 46.1,42.16 48.9,42.16 v49.66,42.16 49.89,42.39 49.89,43.26 50.01,43.38 LED2.+
  Bottom 0.254: v49.66,42.16 49.66,40.51 47.37,38.23 47.37,31.24 42.32,26.19 42.32,26.16 42.13,25.97 39.24,25.97 39.05,25.78 36.45,25.78 35.62,24.96 35.62,23.43 31.75,19.56 25.91,19.56 v25.78,19.68 23.11,19.68 22.61,20.19 19.05,20.19 17.65,18.8 5.08,18.8 J4.5
ENABLE_1  (via drill 0.38)
  Top 0.254: v11.94,24.13 11.94,26.75 12.37,27.18 15.11,27.18 15.62,27.69 15.62,28.96 16.38,29.72 21.72,29.72 22.48,29.72 v23.37,30.61 22.99,30.99 R5.2 | IC1.P$2 21.02,42.15 v20.64,41.77
  Top 0.305: IC3.25 12.31,24.5 v11.94,24.13
  Bottom 0.254: J4.7 11.43,24.64 v11.94,24.13 | v23.37,30.61 22.73,30.61 20.7,32.64 20.7,34.29 20.07,34.93 18.87,34.93 18.19,35.61 18.19,39.98 18.16,40.01 18.16,41.02 18.91,41.77 v20.64,41.77
ENABLE_2  (via drill 0.38)
  Top 0.254: v18.29,20.7 18.29,18.16 18.9,17.55 IC3.35 18.9,14.58 R6.2 | IC2.P$2 36.31,42.15 v35.94,41.78
  Bottom 0.254: J5.5 3.05,20.83 4.95,20.83 6.48,19.3 16.89,19.3 v18.29,20.7 28.7,20.7 29.34,20.07 31.5,20.07 35.05,23.62 35.05,26.61 36.26,27.81 36.26,41.47 v35.94,41.78
GND  (via drill 0.38)
  Top 0.254: 24.88,41.65 24.89,41.65 v24.89,41.15 | 41.65,41.65 41.4,41.65 v41.4,41.15
  Top 0.305: 21.47,41.65 IC1.P$3 24.76,41.65 | 24.76,41.65 24.77,41.66 | v26.92,41.15 IC1.P$18 32,41.15 | 41.66,41.66 41.65,41.65 IC2.P$3 37.85,41.65 | IC2.P$29 IC2.P$18 48.26,41.15 | 24.76,41.65 24.88,41.65
  Top 0.813: 1.78,48.77 JP8.1 J5.12 J4.12 6.22,37.34 | 7.24,55.12 19.05,55.12
  Bottom 0.813: 1.78,50.04 JP8.1 J5.12 J4.12 | 6.86,55.12 19.56,55.12
  other vias: 20.7,46.36 22.1,43.69 28.57,43.69 30.61,43.69 30.99,49.28 20.7,47.75 22.22,46.36 26.92,42.16 24.89,42.16 24.89,40.13 26.92,40.13 28.45,33.53 30.99,33.53 33.27,33.53 23.75,33.53 41.4,42.16 43.43,42.16 43.43,40.13 41.4,40.13 37.85,46.23 38.61,43.69 46.23,43.69 47.5,49.53 47.5,48.13 37.21,48.9 37.21,50.16 39.75,33.78 44.51,31.05 50.04,33.53 42.74,31.05 22.1,33.53 46.86,46.74 42.42,42.16 43.43,41.15 42.42,40.13 42.42,41.15 25.91,41.15 25.91,42.16 25.91,40.13 50.04,48.26 51.31,41.91 7.11,35.66 10.87,32.21 47.41,28.41
  pour Top (isolate 0.305, rank 3): 0.25,56.64 0.25,0.25 56.64,0.25 56.64,56.64
  pour Bottom (isolate 0.305, rank 2): 0.25,28.45 0.25,56.64 56.64,56.64 56.64,29.72 52.58,29.72 52.58,28.45 51.31,27.18 33.97,27.18 33.97,28.89 33.59,28.89 33.53,31.5 7.24,31.5 7.24,28.45
M1_OUT1A
  Top 0.305: 26.41,49.9 IC1.P$24
  Top 0.406: 26.41,49.9 26.41,50.54 JP9.2 27.18,52.71 28.45,53.98 J1.2
M1_OUT1B
  Top 0.254: 31.24,42.67 31.22,42.65
  Top 0.305: 31.34,42.78 31.24,42.67 | 31.22,42.65 IC1.P$21
  Top 0.406: 31.34,42.78 32.51,43.94 32.51,51.31 | 32.51,51.31 JP9.1 | J1.1 32.26,53.85 32.51,53.59 32.51,51.31
M1_OUT2A
  Top 0.305: 25.41,49.9 IC1.P$26
  Top 0.406: 25.41,49.9 25.41,51.31 JP9.3 24.64,53.21 J1.3
M1_OUT2B
  Top 0.305: IC1.P$1 21.51,42.65 21.46,42.7
  Top 0.406: 21.46,42.7 19.56,44.6 19.56,48.77 JP9.4 22.1,53.09 J1.4
M2_OUT1A
  Top 0.305: 42.92,49.78 IC2.P$24
  Top 0.406: 42.92,51.31 42.92,49.78 | 42.92,51.31 JP10.2 | J2.2 42.8,53.85 42.92,53.73 42.92,51.31
M2_OUT1B
  Top 0.254: 47.75,42.67 47.73,42.65
  Top 0.305: 47.86,42.78 47.75,42.67 | 47.73,42.65 IC2.P$21
  Top 0.406: 47.86,42.78 48.77,43.69 48.77,50.01 47.77,51 46.53,51 JP10.1 46.23,53.47 J2.1
M2_OUT2A
  Top 0.305: 41.92,49.78 IC2.P$26
  Top 0.406: 41.92,49.78 41.92,50.54 JP10.3 39.5,52.96 J2.3
M2_OUT2B
  Top 0.305: IC2.P$1 37.11,42.65 36.98,42.78
  Top 0.406: 36.98,42.78 36.07,43.69 36.07,51.31 | 36.07,51.31 JP10.4 | 36.07,51.31 36.07,53.34 J2.4
MCLR  (via drill 0.38)
  Top 0.254: IC1.P$12 26.41,33.65 26.42,33.64 26.43,33.64 27.81,32.26 29.08,32.26 31.11,30.23 v31.11,29.59 32.64,29.59 33.4,30.35 40.39,30.35 42.92,32.89 IC2.P$12 | v19.18,18.41 20.32,19.56 20.32,23.75 v20.07,24 20.07,25.65 21.3,26.89 IC3.18 | v37.02,24.32 36.07,23.37 SW2.3 34.93,22.73 34.29,23.37 R22.1 | v51.87,28.32 52.71,28.32 J8.1
  Bottom 0.254: v51.87,28.32 51.87,26.59 51.69,26.42 44.07,26.42 42.61,24.96 39.75,24.96 39.56,24.77 37.47,24.77 v37.02,24.32 37.02,23.3 32.26,18.54 27.69,18.54 26.92,17.78 25.65,17.78 24.77,18.67 22.61,18.67 22.1,19.18 19.94,19.18 v19.18,18.41 | v31.11,29.59 30.1,28.57 30.1,26.8 26.67,23.37 20.7,23.37 v20.07,24
MS1  (via drill 0.38)
  Top 0.254: IC1.P$9 24.91,33.04 24.89,33.02 v24.89,32.13 | IC2.P$9 41.42,34.05 39.62,32.26 v32.77,32.26 | IC3.27 17.31,22.9 17.4,22.99 v17.78,22.99
  Bottom 0.254: v24.89,32.13 26.04,32.13 26.29,32.38 27.05,32.38 27.18,32.26 v32.77,32.26 32.8,32.26 33.66,31.41 33.66,29.84 31.11,27.3 31.11,26.29 27.18,22.35 19.43,22.35 19.18,22.61 18.16,22.61 v17.78,22.99
MS2  (via drill 0.38)
  Top 0.254: IC1.P$10 25.41,33.03 25.4,33.02 26.67,31.75 v26.67,31.5 | IC2.P$10 41.92,33.66 39.62,31.37 v31.5,31.37 | IC3.26 17.22,23.7 17.4,23.88 18.54,23.88 v18.92,23.49
  Bottom 0.254: v18.92,23.49 19.05,23.49 19.68,22.86 26.92,22.86 30.61,26.54 30.61,27.56 33.15,30.1 33.15,30.83 32.61,31.37 v31.5,31.37 31.11,31.75 26.92,31.75 v26.67,31.5
MS3  (via drill 0.38)
  Top 0.254: IC1.P$11 25.91,33.4 27.56,31.75 28.32,31.75 v29.59,30.48 | IC2.P$11 42.42,33.27 40.01,30.86 32.64,30.86 v32.26,30.48 | IC3.31 16.31,19.68 15.24,19.68 14.99,19.94 12.32,19.94 v11.05,21.21
  Bottom 0.254: v32.26,30.48 v29.59,30.48 29.59,27.05 26.42,23.88 21.46,23.88 20.45,24.89 19.68,24.89 19.18,24.38 18.54,24.38 18.03,23.88 17.4,23.88 16.89,23.37 16.89,22.1 15.62,20.83 11.43,20.83 v11.05,21.21
N$1
  Top 0.254: LED2.- R16.2
N$2
  Top 0.254: D2.- 45.26,16.09 45.24,16.11 | 47.6,16.46 48.01,16.46 F1.1
  Top 0.406: D3.- 45.24,16.11 | D2.- 46.65,16.09 47.02,16.46 47.6,16.46
N$3
  Top 0.254: C2.1 20.32,39.24 22.22,41.15 IC1.P$4
N$4
  Top 0.254: R13.2 R14.1 R18.1
N$5
  Top 0.254: IC1.P$5 22.49,40.65 21.21,39.37 21.21,35.56 20.95,35.31 20.41,35.31 C2.2
N$6
  Top 0.203: 40.49,12.86 J7.P$1
  Top 1.27: D1.+ 40.49,12.86
N$7
  Top 0.254: LED1.- R15.2
N$8
  Top 0.254: USB.- 29.54,2.92 R26.2
N$9
  Top 0.254: R27.1 R23.1 53.59,23.03 53.59,22.35 54.86,21.09 IC4.1
N$10
  Top 0.254: USR.- R25.2
N$11
  Top 0.254: PWR.- R20.2
N$16
  Top 0.254: IC2.P$4 38.61,41.15 36.07,38.61 C4.1
N$17
  Top 0.254: IC2.P$5 39,40.65 36.96,38.61 36.96,35.56 36.7,35.31 C4.2
N$19
  Top 0.254: IC1.P$13 26.91,37.86 27.81,36.96 28.41,36.96 28.41,36.87 R8.1
N$20
  Top 0.254: IC1.P$8 24.41,37.49 C10.1
N$21
  Top 0.254: IC1.P$6 22.75,40.15 22.1,39.5 C5.1
N$31
  Top 0.203: R3.2 24.78,48.3
  Top 0.254: 24.91,48.21 24.78,48.21 24.78,48.3
  Top 0.305: 24.91,48.21 IC1.P$27
N$32
  Top 0.203: R1.2 27.01,48.28 27.01,48.18
  Top 0.254: 26.91,48.08 26.91,48.18 27.01,48.18
  Top 0.305: 26.91,48.08 IC1.P$23
N$36
  Top 0.406: C15.2 48.39,20.56 48.4,20.55 48.44,20.55 | IC4.3 48.44,20.55 | 48.44,20.55 48.06,20.17 F1.2
N$41
  Top 0.254: IC2.P$6 39.26,40.15 38.35,39.24 C6.1
N$43
  Top 0.203: R2.2 44.01,48.67 43.52,48.18
  Top 0.254: 43.42,48.08 43.42,48.18 43.52,48.18
  Top 0.305: 43.42,48.08 IC2.P$23
N$44
  Top 0.203: R4.2 40.83,48.67 41.32,48.18
  Top 0.254: 41.42,48.08 41.42,48.18 41.32,48.18
  Top 0.305: 41.42,48.08 IC2.P$27
N$45
  Top 0.254: IC2.P$8 40.92,37.36 C9.1
N$48
  Top 0.254: IC2.P$13 43.42,37.61 44.07,36.96 44.92,36.96 44.92,36.87 R7.1
N$1234
  Top 0.254: C26.2 13.16,43.79 13.16,43.39 12.63,42.87 12.63,42.77 U5.6 12.32,42.45 12.32,41.1 R29.2
PRG_SW
  Top 0.254: SW1.2 13.84,17.23 14.92,17.23 15.75,16.41 | IC3.30 17.22,20.5 17.53,20.19 17.53,17.47 16.48,16.43 15.77,16.43 15.75,16.41 | 15.75,16.41 R21.1
RA1  (via drill 0.38)
  Top 0.254: v17.91,26.42 19.05,26.42 19.7,27.06 IC3.20
  Bottom 0.254: v17.91,26.42 17.14,25.65 5.97,25.65 4.45,27.18 J4.8
RA2  (via drill 0.38)
  Top 0.254: IC3.21 18.9,28.73 18.41,29.21 16.64,29.21 16.13,28.7 16.13,27.56 v16.51,27.18
  Bottom 0.254: v16.51,27.18 15.49,26.16 7.24,26.16 4.95,28.45 3.05,28.45 J5.8
RA3  (via drill 0.38)
  Top 0.254: IC3.22 17.31,27.9 v17.02,28.19 | J4.9 4.34,29.73 4.33,29.73 9.25,34.65 9.25,39.52 9.65,39.93 10.39,39.93 10.64,40.18 R28.1 10.64,41.38 10.97,41.71 11.23,41.71 11.51,41.99 U5.5
  Bottom 0.254: v17.02,28.19 16.26,28.19 14.73,26.67 7.49,26.67 4.45,29.72 J4.9
RA5  (via drill 0.38)
  Top 0.254: IC3.24 17.37,25.3 v17.78,24.89
  Bottom 0.254: v17.78,24.89 17.53,25.15 5.71,25.15 4.95,25.91 3.05,25.91 J5.7
RB0  (via drill 0.38)
  Top 0.254: IC3.8 23.98,23.7 v22.99,24.69
  Bottom 0.254: JP2.3 11.56,49.66 11.56,36.58 15.37,32.77 18.29,32.77 22.73,28.32 24.94,28.32 26.29,26.97 26.29,25.15 25.53,24.38 23.29,24.38 v22.99,24.69
RB1  (via drill 0.51)
  Top 0.254: IC3.9 25.16,24.5 TP6.P$1
  Bottom 0.254: TP6.P$1 25.4,25.4 25.78,25.78 25.78,26.8 24.77,27.81 22.48,27.81 18.03,32.26 15.11,32.26 11.05,36.32 11.05,48.51 9.52,50.04 JP1.3
  other vias: 24.26,25.4
RB2  (via drill 0.38)
  Top 0.254: IC3.10 26.77,25.3 26.54,25.53 26.54,26.54 27.18,27.18 v27.18,27.43
  Bottom 0.254: v27.18,27.43 26.54,27.43 25.15,28.83 22.99,28.83 18.54,33.27 15.62,33.27 12.07,36.83 12.07,47.62 JP3.3
RB3  (via drill 0.38)
  Top 0.254: IC3.11 27.9,26.75 v28.57,27.43
  Bottom 0.254: v28.57,27.43 27.69,28.32 26.42,28.32 25.4,29.34 23.24,29.34 18.8,33.78 15.88,33.78 12.57,37.08 12.57,47.24 13.97,48.64 15.62,48.64 JP4.3
RB4  (via drill 0.38)
  Top 0.254: IC3.14 24.5,26.96 v24.99,26.47
  Bottom 0.254: JP5.3 6.86,46.99 8.43,45.41 8.43,43.71 9.27,42.88 9.27,37.34 14.86,31.75 17.78,31.75 22.22,27.3 24.15,27.3 v24.99,26.47
RB5  (via drill 0.38)
  Top 0.254: IC3.15 23.7,26.67 v23.49,26.47
  Bottom 0.254: JP6.3 6.86,44.45 8.76,42.55 8.76,37.08 14.61,31.24 17.53,31.24 21.97,26.8 23.16,26.8 v23.49,26.47
RB6  (via drill 0.38)
  Top 0.254: v24.38,17.78 21.46,20.7 21.46,24.38 22.35,25.27 v22.35,25.91 22.35,26.42 22.9,26.96 IC3.16
  Bottom 0.254: v24.38,17.78 24.89,17.27 27.18,17.27 27.94,18.03 32.51,18.03 38.73,24.26 39.81,24.26 40.01,24.45 42.86,24.45 44.2,25.78 52.07,25.78 52.58,26.29 52.58,27.18 53.34,27.94 53.34,32.64 53.72,33.02 53.72,34.67 J8.5 | v22.35,25.91 22.1,25.91 17.27,30.73 14.35,30.73 8.25,36.83 8.25,40.51 6.86,41.91 JP7.3
RB7  (via drill 0.38)
  Top 0.254: v23.11,17.78 20.95,19.94 20.95,25.27 v21.21,25.53 21.21,26.04 22.1,26.92 IC3.17
  Bottom 0.254: v23.11,17.78 24.13,16.76 27.43,16.76 28.19,17.53 32.77,17.53 38.99,23.75 40.07,23.75 40.26,23.94 43.12,23.94 44.32,25.15 52.2,25.15 53.09,26.04 53.09,26.92 53.85,27.69 53.85,32.26 J8.4 | v21.21,25.53 21.21,26.04 17.02,30.23 14.1,30.23 6.86,37.47 JP8.3
RC0  (via drill 0.38)
  Top 0.254: IC3.32 15.14,18.9 14.61,19.43 13.08,19.43 10.16,16.51 v9.65,16.51
  Bottom 0.254: v9.65,16.51 8.76,17.4 4.7,17.4 J4.4
RC2  (via drill 0.38)
  Top 0.254: IC3.36 19.7,17.67 v20.32,18.29 | v30.99,16.64 R14.2
  Bottom 0.254: J5.3 3.05,15.75 5.08,15.75 5.59,16.26 8.38,16.26 9.14,15.49 10.29,15.49 11.56,16.76 18.8,16.76 v20.32,18.29 20.7,18.67 21.72,18.67 22.22,18.16 22.22,17.02 22.99,16.26 27.69,16.26 28.19,16.76 30.86,16.76 v30.99,16.64
RC6  (via drill 0.38)
  Top 0.254: v26.92,14.73 26.67,14.73 26.1,15.3 IC3.44
  Bottom 0.254: v26.92,14.73 26.67,14.99 23.62,14.99 22.61,13.97 21.59,13.97 20.83,14.73 14.86,14.73 12.45,12.32 11.05,12.32 9.4,10.67 3.05,10.67 J5.1
RC7  (via drill 0.38)
  Top 0.254: v28.57,15.88 28.57,18.03 27.83,18.03 IC3.1 | 13.17,14.1 10.71,14.1 10.67,14.06 R12.2 | v13.08,15.37 13.08,14.18 13.17,14.1 | 13.17,14.1 13.17,14.01 R17.1
  Bottom 0.254: v28.57,15.88 28.45,15.75 13.46,15.75 v13.08,15.37 12.45,15.37 10.29,13.21 3.05,13.21 J5.2
RD0  (via drill 0.38)
  Top 0.254: IC3.38 21.3,17.74 v21.34,17.78
  Bottom 0.254: v21.34,17.78 19.81,16.26 11.81,16.26 10.54,14.99 8.89,14.99 8.13,15.75 5.97,15.75 4.7,14.48 J4.3
RD1  (via drill 0.38)
  Top 0.254: v22.1,14.86 IC3.39
  Bottom 0.254: v22.1,14.86 21.72,15.24 14.61,15.24 12.19,12.83 10.8,12.83 9.91,11.94 J4.2
REF_RA0  (via drill 0.38)
  Top 0.254: IC1.P$17 29.46,40.65 v30.35,39.75 | v47.37,39.5 46.99,39.5 45.85,40.64 IC2.P$17 | v18.8,25.53 19.05,25.53 20.5,26.97 IC3.19 20.5,28.88 20.83,29.21 23.49,29.21 v24.51,30.23 | v27.81,30.86 29.08,29.59 29.84,29.59 30.73,28.7 31.5,28.7 31.88,29.08 33.02,29.08 33.78,29.84 34.8,29.84 | 34.8,29.84 v42.42,29.84 | 34.8,29.84 v34.8,28.32 | R11.2 11.76,29.9 10.67,30.99 TP3.1
  Bottom 0.254: v30.35,39.75 34.04,39.75 35.18,38.61 35.18,28.7 v34.8,28.32 | v42.42,29.84 45.21,29.84 46.86,31.5 46.86,38.99 v47.37,39.5 | v18.8,25.53 18.8,27.69 17.4,29.08 16.38,29.08 14.48,27.18 11.79,27.18 | 11.79,27.18 7.75,27.18 5.97,28.96 5.97,29.97 4.95,30.99 3.05,30.99 J5.9 | v24.51,30.23 27.18,30.23 v27.81,30.86 | TP3.1 10.67,30.99 11.81,29.84 11.81,27.2 11.79,27.18
SLEEP_1
  Top 0.254: IC1.P$14 27.41,38.12 27.56,37.97 29.08,37.97 30.1,36.96 30.99,36.96 R9.2
SLEEP_2
  Top 0.254: IC2.P$14 44.7,37.97 45.59,37.97 46.61,36.96 47.5,36.96 R10.2
STEP_1  (via drill 0.38)
  Top 0.254: v30.99,21.46 29.84,20.32 28.96,20.32 28.78,20.5 IC3.4 | IC1.P$16 29.07,40.15 29.34,39.88 29.34,39.37 29.97,38.73 v31.24,38.73
  Bottom 0.254: v31.24,38.73 32.77,38.73 33.15,39.12 33.91,39.12 34.67,38.35 34.67,29.34 33.91,28.57 33.91,24 31.37,21.46 v30.99,21.46 30.86,21.46 30.23,22.1 27.69,22.1 27.3,21.72 19.3,21.72 18.92,22.1 17.65,22.1 15.88,20.32 8,20.32 4.95,23.37 3.05,23.37 J5.6
STEP_2  (via drill 0.38)
  Top 0.254: v49.02,38.61 47.12,38.61 45.58,40.15 IC2.P$16 | IC3.2 26.64,18.9 v26.42,18.67
  Bottom 0.254: v49.02,38.61 47.88,37.47 47.88,30.99 42.57,25.68 42.57,25.65 42.38,25.46 39.5,25.46 39.31,25.27 36.7,25.27 36.13,24.7 36.13,23.18 32,19.05 26.8,19.05 v26.42,18.67 25.53,18.67 25.02,19.18 22.86,19.18 22.35,19.68 19.3,19.68 17.91,18.29 3.05,18.29 J5.4
USB_LED  (via drill 0.38)
  Top 0.254: IC3.41 23.7,13.39 25.4,11.68 v25.91,11.68 | v32.38,3.94 31.81,4.51 31.08,4.51 31.01,4.45 USB.+
  Bottom 0.254: v25.91,11.68 30.86,11.68 32.26,10.29 32.26,3.94 v32.38,3.94
USR_LED  (via drill 0.38)
  Top 0.254: IC3.40 22.9,13.42 v25.91,10.41 | v22.1,3.05 22.1,4.01 22.5,4.42 23.36,4.42 23.36,4.36 USR.+
  Bottom 0.254: v25.91,10.41 25.91,6.86 v22.1,3.05
V+  (via drill 0.38, 0.51)
  Top 0.254: v38.35,33.72 C6.2 | 24.41,44.96 C7.1 | 27.41,44.96 C8.1 | C5.2 22.1,35.18 20.83,33.91 v19.81,33.91 | v40.07,26.92 40.07,26.91 | D2.+ 45.8,19.4 | R13.1 32.73,15.33 33.49,15.33 35.38,17.22 37.77,17.22 39.35,18.8 39.62,18.8 40.49,19.66 D1.-
  Top 0.305: IC1.P$28 24.41,44.96 24.41,45.7 v23.88,46.23 | IC1.P$22 27.41,44.96 27.41,45.7 v27.94,46.23 | 40.92,44.96 40.92,45.7 v40.39,46.23 | 40.92,44.96 IC2.P$28 | 40.92,44.96 C11.1 | 43.92,44.96 43.92,45.57 v44.58,46.23 | 43.92,44.96 IC2.P$22 | 43.92,44.96 C12.1 | U1.1 18.62,43.48 18.47,43.64 18.24,43.64 18.03,43.84 C21.2
  Top 0.406: v30.61,47.5 30.1,47.5 28.83,46.23 v27.94,46.23 | v40.39,46.23 39.5,46.23 38.23,47.5 v37.59,47.5 | 40.49,22.82 43.63,22.82 45.8,20.65 45.8,19.4
  Top 0.61: v17.42,42.11 18.62,42.11 U1.1
  Top 0.813: v40.07,26.92 40.07,28.4 C14.+ | D1.- 40.49,22.82 40.49,26.49 40.07,26.91
  Bottom 0.254: v19.81,33.91 19.43,33.91 19.05,34.29 18.24,34.29 17.42,35.1 v17.42,42.11
  Bottom 0.406: v27.94,46.23 v23.88,46.23 | v40.39,46.23 v44.58,46.23
  Bottom 0.61: v37.59,47.5 34.54,47.5 v30.61,47.5 28.32,49.78 20.65,49.78 17.42,46.56 v17.42,42.11
  Bottom 0.813: 38.23,33.53 38.23,42.42 34.54,46.1 34.54,47.5 | 38.23,33.53 38.23,28.77 v40.07,26.92 | v38.35,33.72 38.35,33.66 38.23,33.53
VBUS  (via drill 0.35, 0.38)
  Top 0.254: R12.1 10.67,10.64 v13.18,8.13 v13.18,8.12 13.18,7.22 13.18,6.86 J3.VBUS | 43.61,19.4 D3.+
  Top 0.406: v43.61,21.08 43.61,19.4
  Bottom 0.406: v43.61,21.08 35.1,12.57 24,12.57 19.56,8.13 v13.18,8.13
VCAP
  Top 0.305: IC3.23 14.44,26.1 14.25,25.91 C13.2

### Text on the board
Top: schmalzhaus.com/EBB | EiBot | Board
Bottom: 6/25/2020
tPlace: GND | GND | 5V | 5V | B1 | B0 | B2 | B3 | GND | B4 | MOTOR1 | DIR1 | MOTOR2 | DIR2 | B5 | 3.3V | B6 | B7 | GND | 3.3V | TP3 | 5V | schmalzhaus.com/EBB | A0 | A3 | CURRENT | 3.3V | A2 | A1 | ADJ | ICSP | A5 | E0 | D6 | D7 | C1 | D5 | D4 | C0 | PRG | RST | C2 | D0 | C7 | D1 | C6 | GND | 9-25VDC | J5 | J4 | EBB | v2.6 | EiBot | Board | PWR | IN | GND | USR | USB
bPlace: GND | 5V | GND | 5V | B1 | B0 | B2 | B3 | B5 | B4 | GND | Arm | Pen | MOTOR 1 | MOTOR 2 | B6 | Servos | 3.3V | B7 | GND | GND | 3.3V | 3.3V | EiBotBoard | PGC(RB6) | 5V | 5V | PGD(RB7) | A0 | A3 | Released under Creative | ICSP | GND | Commons V3.0 Attribution | A2 | A1 | Licence by SchmalzHaus | 3.3V | A5 | E0 | MCLR | D6 | D7 | C1 | D5 | D4 | C0 | C2 | D0 | C7 | D1 | C6 | GND | IO PINS | J5 | J4 | for more information see: | www.schmalzhaus.com/EBB

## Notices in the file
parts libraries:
SparkFun-PowerSymbols: Licensing: Creative Commons ShareAlike 4.0 International - https://creativecommons.org/licenses/by-sa/4.0
